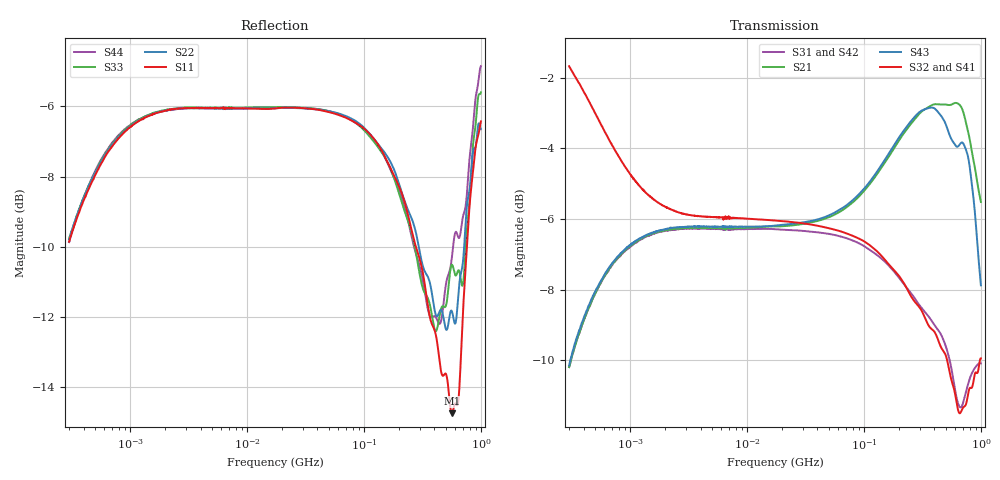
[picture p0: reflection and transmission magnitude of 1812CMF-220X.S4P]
!s-Parameter Generated by FASTRON Sdn. Bhd.
!FASTRON P/N : 1812CMF-220X
!Keysight Technologies: E5071C_MY46733604_B.14.02
!Date: Mon Mar 09 13:16:57 2026
!Version  :Rev00  Mon Mar 09 13:16:57 2026
!Data & Calibration Information:
!Freq	S11:SOLT4(ON)	S12:SOLT4(ON)	S13:SOLT4(ON)	S14:SOLT4(ON)
!	S21:SOLT4(ON)	S22:SOLT4(ON)	S23:SOLT4(ON)	S24:SOLT4(ON)
!	S31:SOLT4(ON)	S32:SOLT4(ON)	S33:SOLT4(ON)	S34:SOLT4(ON)
!	S41:SOLT4(ON)	S42:SOLT4(ON)	S43:SOLT4(ON)	S44:SOLT4(ON)
!PortZ  Port1:50+j0  Port2:50+j0  Port3:50+j0  Port4:50+j0
!When reading reference impedance value at option line is always used.
! Remarks : This data is being provided solely for informational purposes.
# Hz S dB R 50
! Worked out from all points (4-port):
!   1601 points, 300 kHz to 1 GHz, reference 50 ohm
!   strongest paths, dB at 300 kHz, 2.303 MHz, 17.55 MHz, 132.8 MHz, 1 GHz:
!     S32: -1.7, -5.7, -6.0, -6.9, -9.9
!     S41: -1.6, -5.8, -6.0, -6.9, -10.2
!     S43: -10.1, -6.2, -6.2, -4.6, -7.9
!     S21: -10.2, -6.3, -6.2, -4.7, -5.5
!     S31: -10.2, -6.3, -6.3, -7.0, -10.1
!     S42: -10.2, -6.3, -6.3, -7.1, -10.3
!   lowest |S11| = -14.7 dB at 562.9 MHz (marker M1), VSWR 1.45, Z = 72.2 - j3.11 ohm
!   |S11| at or under -10 dB: 277.9 MHz to 759.5 MHz (481.6 MHz wide, 92.8 % of centre)
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300000  -9.85 44.8  -10.21 49.5  -10.22 -130.7  -1.73 -16.9
        -10.19 49.4  -9.79 45.6  -1.68 -17.3  -10.30 -130.5
        -10.19 -130.8  -1.67 -17.3  -9.77 45.5  -10.28 49.7
        -1.63 -17.5  -10.18 -130.9  -10.14 49.2  -9.87 46.7
1519487  -6.24 12.9  -6.40 13.8  -6.41 -166.9  -5.39 -12.8
         -6.42 13.8  -6.24 12.9  -5.36 -12.8  -6.44 -166.8
         -6.44 -166.8  -5.39 -12.8  -6.22 12.9  -6.41 13.9
         -5.41 -12.7  -6.45 -166.8  -6.40 13.9  -6.22 12.8
5.251762e7  -6.18 -10.3  -5.91 6.4  -6.42 164.3  -6.28 -15.7
            -5.92 6.5  -6.15 -9.9  -6.26 -16.3  -6.47 165.3
            -6.43 164.3  -6.28 -16.3  -6.16 -10.8  -5.90 6.6
            -6.26 -15.8  -6.45 165.2  -5.87 6.6  -6.15 -9.4
2.162177e8  -8.59 -34.4  -3.59 6.9  -7.80 121.6  -7.78 -55.1
            -3.60 6.9  -8.58 -32.2  -7.76 -56.7  -7.82 125.1
            -7.81 121.7  -7.78 -56.6  -8.86 -35.1  -3.54 6.2
            -7.77 -54.9  -7.81 125.2  -3.52 6.1  -8.72 -29.5
3.712352e8  -12.09 -35.0  -2.78 -2.5  -8.83 89.3  -8.85 -86.3
            -2.80 -2.5  -11.12 -30.0  -9.08 -88.3  -8.86 94.3
            -8.83 89.4  -9.09 -88.3  -11.75 -28.1  -2.88 -5.0
            -8.84 -86.5  -8.86 94.1  -2.85 -5.0  -12.00 -23.3
5.62905e8  -14.75 -6.5  -2.75 -12.2  -10.27 50.9  -10.27 -126.2
           -2.76 -12.1  -11.83 -7.9  -10.59 -128.2  -10.08 55.3
           -10.27 50.9  -10.58 -128.3  -10.51 -8.3  -3.78 -14.9
           -10.31 -126.3  -10.09 55.3  -3.75 -15.0  -10.35 0.7
1e9  -6.43 22.6  -5.51 -27.4  -10.08 -17.4  -10.21 160.3
     -5.52 -27.2  -6.65 8.9  -9.96 149.3  -10.35 -24.3
     -10.08 -17.4  -9.94 149.1  -5.60 2.0  -7.90 -21.4
     -10.24 160.0  -10.33 -24.3  -7.87 -21.2  -4.86 5.1
